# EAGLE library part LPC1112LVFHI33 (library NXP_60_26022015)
32-bit ARM Cortex-M0 microcontroller The LPC111xLV/LPC11xxLVUK is an ARM Cortex-M0-based, low-cost 32-bit MCU family, designed for 8/16-bit microcontroller applications, offering performance, low power, simple instruction set and memory addressing together with reduced code size compared to existing 8/16-bit architectures. The LPC111xLV/LPC11xxLVUK operate at CPU frequencies of up to 50 MHz. The peripherals of the LPC111xLV/LPC11xxLVUK include up to 32 kB of flash memory, up to 8 kB of SRAM data memory, a Fast-mode Plus I 2 C-bus interface, one SSP/SPI interface, one UART, four general-purpose counter/timers, an 8-bit ADC, and up to 27 general-purpose I/O pins. MK - Datasheet available on www.nxp.com
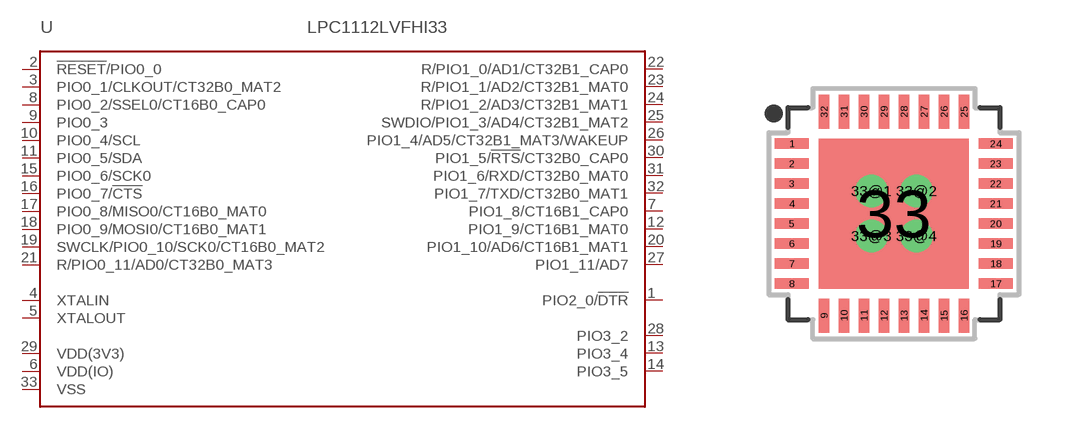
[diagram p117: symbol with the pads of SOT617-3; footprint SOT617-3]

Designator prefix U

## LPC1112LVFHI33  [SOT617-3]
1  PIO2_0/!DTR!
2  !RESET!/PIO0_0
3  PIO0_1/CLKOUT/CT32B0_MAT2
4  XTALIN  in
5  XTALOUT  out
6  VDD(IO)  pwr
7  PIO1_8/CT16B1_CAP0
8  PIO0_2/SSEL0/CT16B0_CAP0
9  PIO0_3
10  PIO0_4/SCL
11  PIO0_5/SDA
12  PIO1_9/CT16B1_MAT0
13  PIO3_4
14  PIO3_5
15  PIO0_6/SCK0
16  PIO0_7/!CTS!
17  PIO0_8/MISO0/CT16B0_MAT0
18  PIO0_9/MOSI0/CT16B0_MAT1
19  SWCLK/PIO0_10/SCK0/CT16B0_MAT2
20  PIO1_10/AD6/CT16B1_MAT1
21  R/PIO0_11/AD0/CT32B0_MAT3
22  R/PIO1_0/AD1/CT32B1_CAP0
23  R/PIO1_1/AD2/CT32B1_MAT0
24  R/PIO1_2/AD3/CT32B1_MAT1
25  SWDIO/PIO1_3/AD4/CT32B1_MAT2
26  PIO1_4/AD5/CT32B1_MAT3/WAKEUP
27  PIO1_11/AD7
28  PIO3_2
29  VDD(3V3)  pwr
30  PIO1_5/!RTS!/CT32B0_CAP0
31  PIO1_6/RXD/CT32B0_MAT0
32  PIO1_7/TXD/CT32B0_MAT1
33  VSS  pwr

## Footprint SOT617-3 (pad centres in mm)
SOT617-3 HVQFN32: plastic thermal enhanced very thin quad flat package; no leads; 32 terminals; body 5 x 5 x 0.85 mm JEDEC: MO-220 IEC: -- JEITA: --
smd 0.85 x 0.27: 1 -2.55,1.75; 2 -2.55,1.25; 3 -2.55,0.75; 4 -2.55,0.25; 5 -2.55,-0.25; 6 -2.55,-0.75; 7 -2.55,-1.25; 8 -2.55,-1.75; 17 2.55,-1.75; 18 2.55,-1.25; 19 2.55,-0.75; 20 2.55,-0.25; 21 2.55,0.25; 22 2.55,0.75; 23 2.55,1.25; 24 2.55,1.75
smd 0.27 x 0.85: 9 -1.75,-2.55; 10 -1.25,-2.55; 11 -0.75,-2.55; 12 -0.25,-2.55; 13 0.25,-2.55; 14 0.75,-2.55; 15 1.25,-2.55; 16 1.75,-2.55; 25 1.75,2.55; 26 1.25,2.55; 27 0.75,2.55; 28 0.25,2.55; 29 -0.25,2.55; 30 -0.75,2.55; 31 -1.25,2.55; 32 -1.75,2.55
smd 3.75 x 3.75: 33 0,0
drill 0.3 pad 0.6: 33@1 -0.562,0.562; 33@2 0.562,0.562; 33@3 -0.562,-0.562; 33@4 0.562,-0.562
